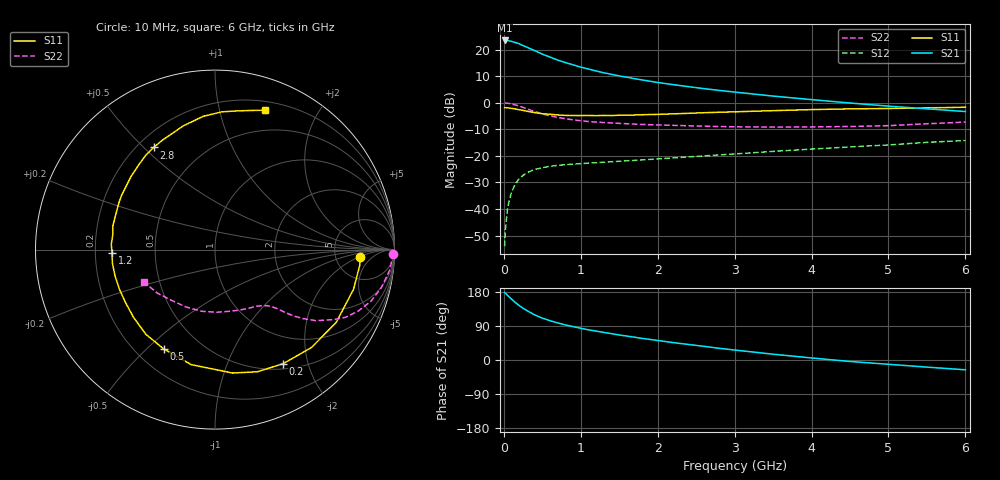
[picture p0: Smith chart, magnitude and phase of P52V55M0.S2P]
! SIEMENS Small Signal Semiconductors
! BFP183
! Si NPN RF Bipolar Junction Transistor in SOT143
! VCE = 2.5 V  IC = 5 mA
! Common Emitter S-Parameters:  March  1996
# GHz  S  MA  R  50
!  f  S11  S21  S12  S22
! GHz  MAG  ANG  MAG  ANG  MAG  ANG  MAG  ANG
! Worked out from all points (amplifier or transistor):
!   36 points, 10 MHz to 6 GHz, reference 50 ohm
!   highest |S21| = 23.5 dB at 10 MHz (marker M1)
!   |S21| within 3 dB of that: start of sweep to 336.5 MHz
!   unconditionally stable (mu >= 1): 1.55 GHz to 5.721 GHz
!   at 250 MHz: K = 0.20, MSG = 24.4 dB, |S12| = -27.4 dB
!   at 1.4 GHz: K = 0.95, MSG = 16.5 dB, |S12| = -22.2 dB
!   at 6 GHz: K = 0.95, MSG = 5.5 dB, |S12| = -14.2 dB
!   lowest NFmin = 1.15 dB at 450 MHz
!   S11 on the Smith chart (normalised r, x): 10 MHz: 8.97, -2.29; 200 MHz: 0.57, -1.61; 500 MHz: 0.31, -0.57; 1.2 GHz: 0.27, -0.02; 2.8 GHz: 0.26, +0.54; 6 GHz: 0.28, +1.39
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0.01  0.8106 -3.1  14.93 178.2  0.002 86.1  0.9922 -1.3
0.02  0.8111 -6.3  14.87 176.5  0.0041 85.8  0.989 -2.6
0.05  0.8029 -16.0  14.9 170.1  0.0109 82.8  0.9812 -6.5
0.1  0.7877 -31.0  14.32 160.7  0.021 73.6  0.9513 -12.8
0.15  0.7656 -45.5  13.65 151.7  0.0297 66.6  0.9145 -18.4
0.2  0.7401 -59.2  12.93 143.5  0.0375 61.0  0.8678 -23.3
0.25  0.7203 -70.9  11.94 136.4  0.0429 55.8  0.819 -27.4
0.3  0.6947 -81.9  11.15 130.4  0.0485 51.7  0.7702 -30.4
0.4  0.6544 -101.6  9.624 119.1  0.0555 44.2  0.6869 -35.2
0.5  0.6231 -117.2  8.259 110.6  0.0601 39.3  0.6186 -38.3
0.6  0.6092 -129.2  7.259 103.8  0.0638 36.2  0.5694 -40.3
0.7  0.5905 -140.1  6.362 97.8  0.0664 33.9  0.5317 -41.6
0.9  0.5764 -157.5  5.188 88.1  0.0702 31.4  0.4779 -43.5
1.1  0.5768 -172.2  4.324 79.6  0.0734 30.1  0.4449 -45.5
1.2  0.574 -178.0  3.971 76.2  0.0746 29.6  0.434 -46.4
1.7  0.5896 157.6  2.849 60.1  0.0825 30.3  0.3972 -52.4
2.2  0.62 139.2  2.2 46.0  0.0917 31.0  0.3766 -60.2
2.8  0.6642 121.0  1.712 30.9  0.1046 31.4  0.3576 -72.2
3.5  0.7115 104.4  1.339 15.3  0.1217 30.4  0.349 -88.6
4.5  0.7683 87.2  0.991 -3.9  0.1478 26.4  0.3584 -117.1
5.5  0.8015 75.3  0.771 -18.8  0.1802 21.5  0.4031 -143.1
6  0.8257 70.1  0.685 -25.9  0.1951 17.5  0.4335 -155.2
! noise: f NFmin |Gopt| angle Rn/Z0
0.45  1.15  0.25  40  0.26
0.9  1.2  0.25  93  0.22
1.8  1.95  0.32  170  0.13
